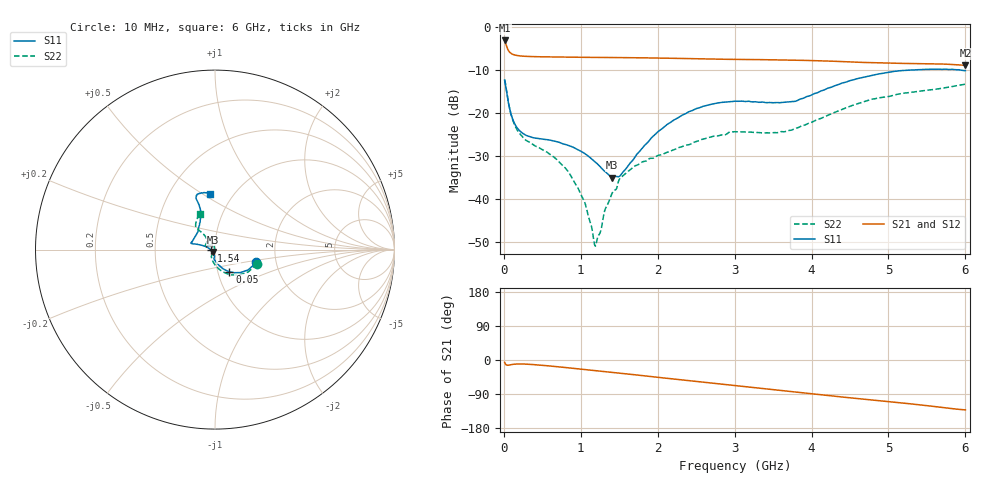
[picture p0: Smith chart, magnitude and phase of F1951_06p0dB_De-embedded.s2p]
! Integrated Device Technology
! Corporate Headquarters
! 6024 Silver Creek Valley Road
! San Jose, CA 95138  USA
! Phone:  1-408-284-8200
! Toll Free:  1-800-223-1366
! Webpage:  http://www.idt.com/
! Timing and RF Division
! 515 Groton Road, Suite 102
! Westford, MA 01886-6024
! Device:  F1951
! Description: 6-bit 0.5 dB Digital Step Attenuator
! Frequency:  100.0 -  4000.00 MHz
! Package:  4x4 mm Thin QFN Plastic Package: 24 pin
! Ports:  2 RF, 6 DC
!  Pin  1  = NC
!  Pin  2  = RF1  =  Port 1
!  Pin  3  = GND
!  Pin  4  = NC
!  Pin  5  = Serial Data Out (SDO)
!  Pin  6  = NC
!  Pin  7  = Reset Bar ( RSTb)
!  Pin  8  = Clock (CLK)
!  Pin  9  = Chip Select Bar (CSb)
!  Pin 10  = NC
!  Pin 11  = Serial Data In (SDI)
!  Pin 12  = NC
!  Pin 13  = NC
!  Pin 14  = VDD
!  Pin 15  = NC
!  Pin 16  = GND
!  Pin 17  = RF2  =  Port 2
!  Pin 18  = NC
!  Pin 19  = GND
!  Pin 20  = GND
!  Pin 21  = GND
!  Pin 22  = GND
!  Pin 23  = GND
!  Pin 24  = GND
! State:  12
! Atten State:  6.0 dB
! Voltage:  +3.30 Volts
! Current:  0.473 mA
! Data:  The device was measured on a F195X evaluation board which has
!  individual transmission lines to the RF pins.  Data was collected
!  de-embedded using a Automatic Fixture Removal [AFR] (Keysight Technologies).
!  The reference plane is the edge of the package pin.
! Misc:  Lot Code  1225BCA
!  Action Tracker AT0399
! Date Measured:  2018-09-13
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# GHz S dB R 50
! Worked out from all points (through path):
!   600 points, 10 MHz to 6 GHz, reference 50 ohm
!   highest |S21| = -3.04 dB at 10 MHz (marker M1); lowest = -8.8 dB at 6 GHz (marker M2)
!   group delay of S21, straight-line fit = 59 ps
!   lowest |S11| = -35.0 dB at 1.41 GHz (marker M3), VSWR 1.04, Z = 48.7 - j1.22 ohm
!   |S11| at or under -10 dB: start of sweep to 5.24 GHz; 5.95 GHz to end of sweep
!   |S22| runs from -51.1 to -12.1 dB; largest |S21 - S12| = 0.0007
!   S11 on the Smith chart (normalised r, x): 10 MHz: 1.58, -0.24; 50 MHz: 1.14, -0.29; 1.54 GHz: 0.96, -0.01; 6 GHz: 0.78, +0.54
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0.01  -12.33 -17.2  -3.04 -6.1  -3.04 -6.1  -12.11 -18.5
0.05  -16.63 -57.0  -5.08 -13.9  -5.08 -13.9  -16.51 -63.6
0.09  -20.02 -72.1  -6.01 -12.3  -6.01 -12.3  -20.08 -83.2
0.13  -22.08 -80.4  -6.37 -11.2  -6.37 -11.1  -22.29 -94.4
0.24  -24.63 -91.6  -6.69 -10.5  -6.69 -10.5  -25.50 -110.2
0.78  -27.23 -94.9  -6.92 -19.4  -6.92 -19.4  -32.47 -119.9
1.01  -28.98 -94.2  -6.97 -24.1  -6.97 -24.1  -39.31 -120.0
1.06  -29.53 -95.9  -6.98 -25.2  -6.98 -25.1  -41.27 -121.9
1.19  -31.47 -102.5  -6.99 -27.8  -6.99 -27.9  -51.06 177.6
1.22  -31.91 -105.1  -6.99 -28.5  -7.00 -28.5  -49.01 151.7
1.32  -33.68 -117.8  -7.00 -30.7  -7.01 -30.7  -42.31 111.2
1.41  -35.03 -135.2  -7.02 -32.6  -7.02 -32.6  -38.61 101.9
1.54  -33.94 -166.7  -7.05 -35.3  -7.05 -35.3  -34.75 103.0
1.7  -30.38 170.9  -7.07 -38.9  -7.07 -38.9  -32.36 106.8
2.01  -24.24 162.1  -7.15 -45.8  -7.15 -45.8  -29.84 123.0
2.49  -19.02 164.1  -7.29 -56.4  -7.29 -56.4  -26.69 151.4
3.01  -17.21 165.4  -7.45 -67.6  -7.45 -67.6  -24.33 161.8
3.56  -17.55 147.4  -7.56 -79.6  -7.57 -79.6  -24.56 143.5
4.01  -15.67 121.3  -7.73 -89.5  -7.73 -89.4  -22.08 127.6
4.55  -12.20 109.7  -8.07 -100.9  -8.07 -100.8  -18.08 128.4
5.01  -10.45 110.3  -8.34 -110.0  -8.34 -110.0  -16.10 130.7
6  -10.08 95.5  -8.83 -131.7  -8.83 -131.7  -13.24 113.2
